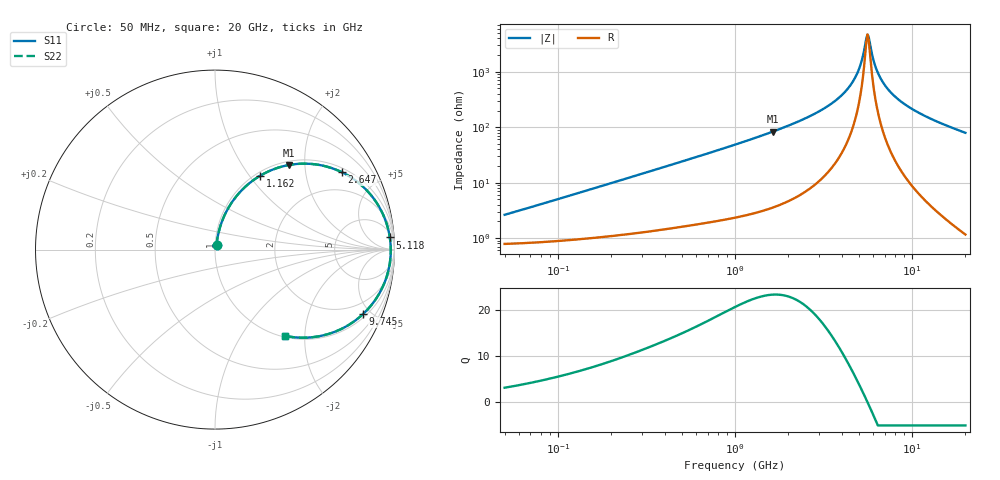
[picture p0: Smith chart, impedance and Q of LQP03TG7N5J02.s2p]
!Murata Part Number: LQP03TG7N5J02
!These Parameters are Measured in Series Mode Connection
!  o--[Z]--o
!Port1  Port2
!  o-------o
!Freq. Start=50[MHz] Stop=20[GHz], 401[Steps]
# Hz S RI R 50
!Freq.(Hz) S11(Real) S11(Imag) S21(Real) S21(Imag) S12(Real) S12(Imag) S22(Real) S22(Imag)
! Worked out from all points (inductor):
!   401 points, 50 MHz to 20 GHz, reference 50 ohm
!   read as one part in series: L = 7.96 nH near 51.52 MHz
!   highest Q = 23.5 at 1.639 GHz (marker M1), where L = 8.1 nH
!   self-resonance near 5.599 GHz
!   S11 on the Smith chart (normalised r, x): 50 MHz: 1.02, +0.05; 1.162 GHz: 1.05, +1.13; 2.647 GHz: 1.16, +3.16; 5.118 GHz: 9, +26; 9.745 GHz: 1.19, -4.48; 20 GHz: 1.02, -1.58
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5e7  0.00838 0.0247  0.9916 -0.0247  0.9916 -0.0247  0.00838 0.0247
1.364002e8  0.0139 0.0655  0.9861 -0.0655  0.9861 -0.0655  0.0139 0.0655
3.721004e8  0.0434 0.1686  0.9566 -0.1686  0.9566 -0.1686  0.0434 0.1686
6.476653e8  0.101 0.2734  0.899 -0.2734  0.899 -0.2734  0.101 0.2734
1e9  0.2009 0.3773  0.7991 -0.3773  0.7991 -0.3773  0.2009 0.3773
1.161586e9  0.2531 0.4126  0.7469 -0.4126  0.7469 -0.4126  0.2531 0.4126
1.639343e9  0.4142 0.4717  0.5858 -0.4717  0.5858 -0.4717  0.4142 0.4717
2.647493e9  0.7051 0.432  0.2949 -0.432  0.2949 -0.432  0.7051 0.432
2.728004e9  0.7233 0.4228  0.2767 -0.4228  0.2767 -0.4228  0.7233 0.4228
3.415248e9  0.8477 0.3279  0.1523 -0.3279  0.1523 -0.3279  0.8477 0.3279
4.087748e9  0.923 0.2229  0.077 -0.2229  0.077 -0.2229  0.923 0.2229
4.677679e9  0.9599 0.1319  0.0401 -0.1319  0.0401 -0.1319  0.9599 0.1319
5.117541e9  0.974 0.0675  0.026 -0.0675  0.026 -0.0675  0.974 0.0675
5.515528e9  0.979 0.0126  0.021 -0.0126  0.021 -0.0126  0.979 0.0126
5.683258e9  0.9793 -0.00946  0.0207 0.00946  0.0207 0.00946  0.9793 -0.00946
6.125241e9  0.9755 -0.0645  0.0245 0.0645  0.0245 0.0645  0.9755 -0.0645
6.406762e9  0.9702 -0.0972  0.0298 0.0972  0.0298 0.0972  0.9702 -0.0972
6.802353e9  0.9598 -0.1401  0.0402 0.1401  0.0402 0.1401  0.9598 -0.1401
7.442007e9  0.9369 -0.202  0.0631 0.202  0.0631 0.202  0.9369 -0.202
9.745021e9  0.8234 -0.3604  0.1766 0.3604  0.1766 0.3604  0.8234 -0.3604
1.375312e10  0.6159 -0.4746  0.3841 0.4746  0.3841 0.4746  0.6159 -0.4746
2e10  0.3873 -0.4799  0.6127 0.4799  0.6127 0.4799  0.3873 -0.4799
